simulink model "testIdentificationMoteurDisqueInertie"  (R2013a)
settings: Solver=ode45  StartTime=0  StopTime=1  FixedStep=1e-3  MaxStep=SimParam.Te  RelTol=1e-4  AbsTol=1e-4
PreLoadFcn:
  | warning('off','sm:sli:setup:compile:LocalSolverNotSupported')
model workspace (MAT data in the model file):
  handle : class17 (value not decoded)
  handle : class17 (value not decoded)
undefined symbols (not defined in the file or in its folder): SimParam

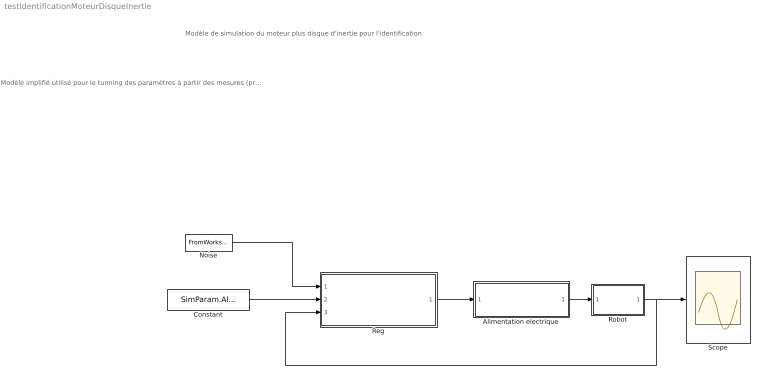
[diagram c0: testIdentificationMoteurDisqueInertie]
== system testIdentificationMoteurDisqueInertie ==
  note: Modèle de simulation du moteur plus disque d'inertie pour l'identification
  note: Modèle implifié utilisé pour le tunning des paramètres à partir des mesures (prbs) effectuée sur le robot (Idem testIdentificationMoteur mais avec un élèment flexible dans le moteur) - Régulateur PID simple avec quantification codeur - Alimentation éléctrique modélisée par une fonction de transfert d'ordre deux avec delais (delais du contrôle) - Méchanique comprennant uniquement un modèle du moteur (inertie + frottement + 1ddl flexible en torsion) + frottement sec - Signaux d'exitation comprennant un bruit blanc et un signal cyclique (PRBS)
  Alimentation electrique : Subsystem
  Constant : Constant  Value=SimParam.Alpha_c
  Noise : FromWorkspace  VariableName=SimIn  SampleTime=SimParam.Te  Interpolate=off  OutputAfterFinalValue=Holding final value
  Reg : Subsystem
  Robot : Subsystem
  Scope : Scope
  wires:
  Noise/1 -> Reg/1(Noise)
  Alimentation electrique/1(Torque_out) -> Robot/1(Tmotor)
  Robot/1(Out1) -> Scope/1, Reg/3(Alpha)
  Reg/1(Torque) -> Alimentation electrique/1(Torque_in)
  Constant/1 -> Reg/2(Alpha_c)

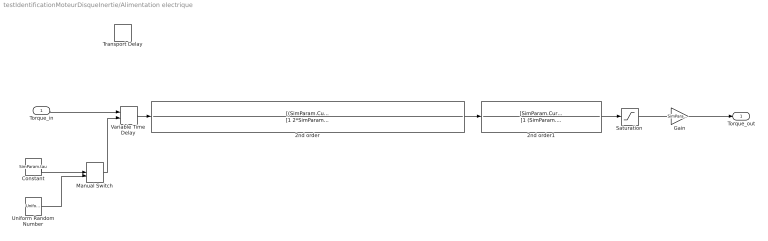
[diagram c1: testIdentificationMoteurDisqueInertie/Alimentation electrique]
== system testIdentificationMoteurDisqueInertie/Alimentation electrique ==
  Torque_in : Inport
  2nd order : TransferFcn  Numerator=[(SimParam.CurrentLoop.f0*2*pi)^2]  Denominator=[1 2*SimParam.CurrentLoop.Cr*(SimParam.CurrentLoop.f0*2*pi) (SimParam.CurrentLoop.f0*2*pi)^2]
  2nd order1 : TransferFcn  Numerator=[SimParam.CurrentLoop.f1*2*pi]  Denominator=[1 (SimParam.CurrentLoop.f1*2*pi)]
  Constant : Constant  Value=SimParam.tau
  Gain : Gain  Gain=SimParam.Grel
  Manual Switch : ManualSwitch  CurrentSetting=0
  Saturation : Saturate  UpperLimit=10  LowerLimit=-10
  Transport Delay : TransportDelay  Commented=on  DelayTime=SimParam.tau
  Uniform Random Number : UniformRandomNumber  Minimum=SimParam.tau-SimParam.Dtau  Maximum=SimParam.tau+SimParam.Dtau  SampleTime=SimParam.Te
  Variable Time Delay : VariableTransportDelay  MaximumDelay=2e-3
  Torque_out : Outport
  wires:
  Saturation/1 -> Gain/1
  Constant/1 -> Manual Switch/1
  Manual Switch/1 -> Variable Time Delay/2
  Uniform Random Number/1 -> Manual Switch/2
  Torque_in/1 -> Variable Time Delay/1
  Variable Time Delay/1 -> 2nd order/1
  2nd order/1 -> 2nd order1/1
  2nd order1/1 -> Saturation/1
  Gain/1 -> Torque_out/1

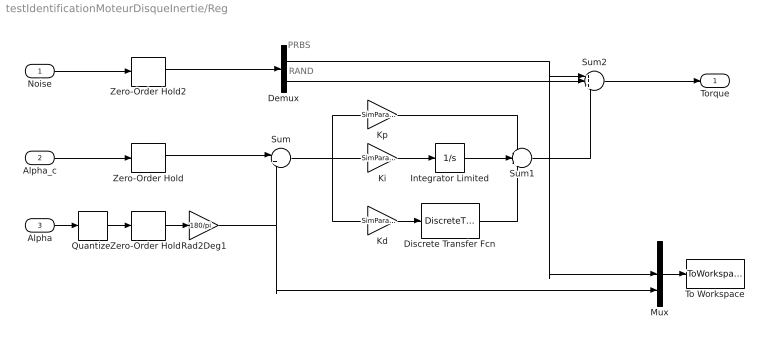
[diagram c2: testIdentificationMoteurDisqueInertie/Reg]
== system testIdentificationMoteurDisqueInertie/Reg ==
  note: RAND
  note: PRBS
  Noise : Inport
  Alpha_c : Inport  Port=2
  Alpha : Inport  Port=3
  Demux : Demux  Outputs=2
  Discrete Transfer Fcn : DiscreteTransferFcn  Numerator=[1 0 -1]  Denominator=[2 0 0]
  Integrator Limited : Integrator  LimitOutput=on  UpperSaturationLimit=1  LowerSaturationLimit=-1
  Kd : Gain  Gain=SimParam.Control.Kd/SimParam.Te
  Ki : Gain  Gain=SimParam.Control.Ki*SimParam.Te
  Kp : Gain  Gain=SimParam.Control.Kp
  Mux : Mux  Inputs=3
  Quantizer : Quantizer  QuantizationInterval=SimParam.CoderResol
  Rad2Deg1 : Gain  Gain=180/pi
  Sum : Sum  Inputs=|+-
  Sum1 : Sum  Inputs=+++
  Sum2 : Sum  Inputs=+++
  To Workspace : ToWorkspace  VariableName=simout  SampleTime=SimParam.Te  SaveFormat=Structure With Time
  Zero-Order Hold : ZeroOrderHold  SampleTime=SimParam.Te
  Zero-Order Hold1 : ZeroOrderHold  SampleTime=SimParam.Te
  Zero-Order Hold2 : ZeroOrderHold  SampleTime=SimParam.Te
  Torque : Outport
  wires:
  Alpha_c/1 -> Zero-Order Hold/1
  Kd/1 -> Discrete Transfer Fcn/1
  Mux/1 -> To Workspace/1
  Zero-Order Hold/1 -> Sum/1
  Alpha/1 -> Quantizer/1
  Quantizer/1 -> Zero-Order Hold1/1
  Noise/1 -> Zero-Order Hold2/1
  Discrete Transfer Fcn/1 -> Sum1/3
  Kp/1 -> Sum1/1
  Sum1/1 -> Sum2/3
  Demux/1 -> Mux/2, Sum2/1
  Sum2/1 -> Torque/1
  Ki/1 -> Integrator Limited/1
  Integrator Limited/1 -> Sum1/2
  Sum/1 -> Ki/1, Kp/1, Kd/1
  Zero-Order Hold1/1 -> Rad2Deg1/1
  Rad2Deg1/1 -> Mux/3, Sum/2
  Demux/2 -> Sum2/2
  Zero-Order Hold2/1 -> Demux/1

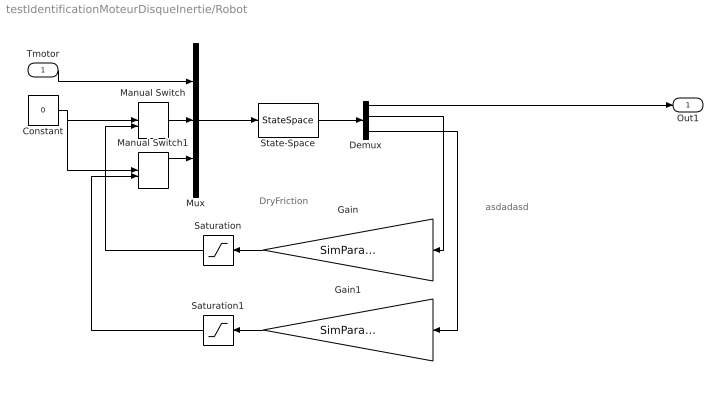
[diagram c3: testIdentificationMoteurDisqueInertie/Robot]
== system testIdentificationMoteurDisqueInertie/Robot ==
  note: asdadasd
  note: DryFriction
  Tmotor : Inport
  Constant : Constant  Value=0
  Demux : Demux
  Gain : Gain  Gain=SimParam.CdmotorSlope
  Gain1 : Gain  Gain=SimParam.CdmotorSlope
  Manual Switch : ManualSwitch  CurrentSetting=0
  Manual Switch1 : ManualSwitch  CurrentSetting=0
  Mux : Mux  Inputs=3
  Saturation : Saturate  UpperLimit=1  LowerLimit=-1
  Saturation1 : Saturate  UpperLimit=1  LowerLimit=-1
  State-Space : StateSpace  A=SimParam.Mec.A  B=SimParam.Mec.B  C=SimParam.Mec.C  D=SimParam.Mec.D
  Out1 : Outport
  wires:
  Gain/1 -> Saturation/1
  Saturation/1 -> Manual Switch/2
  Constant/1 -> Manual Switch/1, Manual Switch1/1
  State-Space/1 -> Demux/1
  Mux/1 -> State-Space/1
  Manual Switch/1 -> Mux/2
  Manual Switch1/1 -> Mux/3
  Demux/2 -> Gain/1
  Gain1/1 -> Saturation1/1
  Saturation1/1 -> Manual Switch1/2
  Demux/4 -> Gain1/1
  Tmotor/1 -> Mux/1
  Demux/1 -> Out1/1
